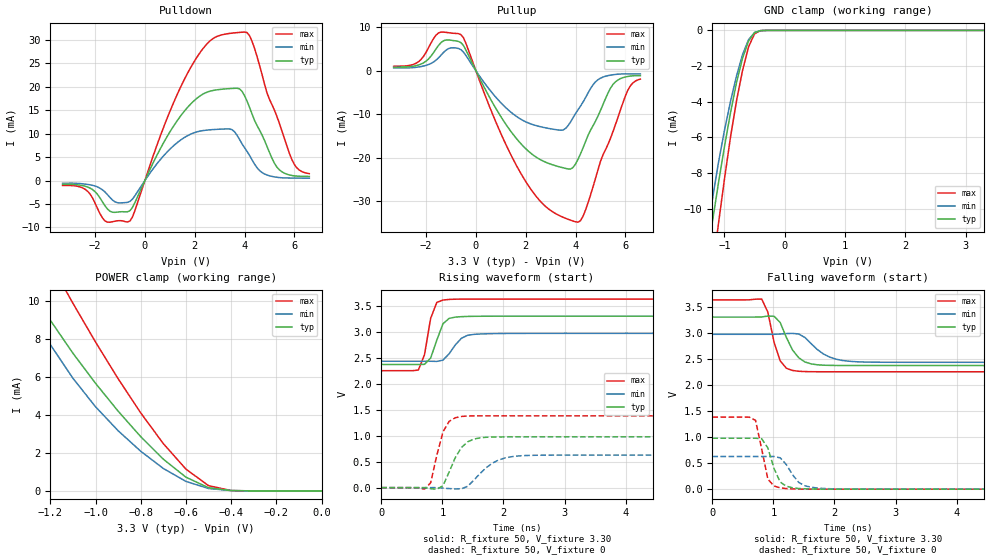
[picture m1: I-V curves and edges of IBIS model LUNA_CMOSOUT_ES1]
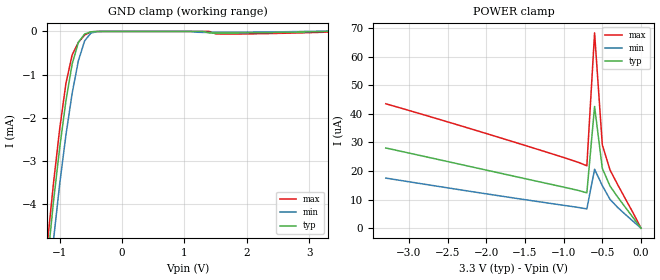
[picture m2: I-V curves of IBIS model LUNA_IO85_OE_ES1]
[IBIS Ver]   3.2
[Comment Char]   |_char
[File name]   sg-9101cga_33v_c.ibs
[File Rev]   1.0
[Date]   2017/11/24 16:18:06
[Source]
[Notes]
[Disclaimer]
This information is for modeling purposes only, and is not guaranteed.
Property of SEIKO EPSON Corp.,
unauthorized reproduction and/or distribution is strictly prohibited.
[Copyright]
Copyright 2017, SEIKO EPSON Corp.
[Component]   SG-9101CGA
Si_location Pin
Timing_location Pin
[Manufacturer]   SEIKO EPSON Corp.
| 2520 PKG
| 2520 PKG
[Package]
R_pkg   238m   NA   NA
L_pkg   2.1n   NA   NA
C_pkg   0.38p   NA   NA
[Pin] signal_name   model_name
1   OE   LUNA_IO85_OE_ES1
2   VSS   GND
3   OUT   LUNA_CMOSOUT_ES1
4   VDD   POWER
| Models and submodels in the file (2): LUNA_CMOSOUT_ES1 (3-state), LUNA_IO85_OE_ES1 (Input)
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[Model]   LUNA_CMOSOUT_ES1
Model_type 3-state
Enable Active-High
Polarity Non-Inverting
Vmeas=1.65
C_comp   2.5p   2.0p   3.0p
[Temperature Range] 25   105   -40
[Voltage Range]   3.30   2.97   3.63
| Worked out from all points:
|   slope of the pulldown table from 0 to 0.495 V, typ, clamps not added: 89.7 ohm
|   slope of the pullup table from 0 to 0.495 V, typ, clamps not added: 88.8 ohm
|   GND clamp passes 1 mA (typ) near -0.64 V on its own axis
|   POWER clamp passes 1 mA (typ) near -0.63 V on its own axis
|   falling waveform, R_fixture 50, V_fixture 3.30: 20-80 % time 249ps typ, 352ps min, 176ps max; typ from 3.3 V to 2.37 V
|   falling waveform, R_fixture 50, V_fixture 0: 20-80 % time 177ps typ, 233ps min, 148ps max; typ from 0.977 V to 0 V
|   rising waveform, R_fixture 50, V_fixture 3.30: 20-80 % time 170ps typ, 222ps min, 143ps max; typ from 2.37 V to 3.3 V
|   rising waveform, R_fixture 50, V_fixture 0: 20-80 % time 249ps typ, 369ps min, 183ps max; typ from 0 V to 0.977 V
[Pullup]
-3.3V     819.1uA    632.4uA    1.02mA
-2.3V     1.324mA    861.7uA    2.085mA
-1.5V     5.824mA    2.966mA    8.695mA
-600mV    6.462mA    4.844mA    8.302mA
900mV     -9.633mA   -6.754mA   -13.14mA
2V        -17.97mA   -11.78mA   -25.53mA
3.5V      -22.37mA   -13.65mA   -33.77mA
4.1V      -20.39mA   -8.97mA    -34.9mA
4.8V      -11.62mA   -2.566mA   -24.81mA
5.5V      -3.173mA   -932.8uA   -14.04mA
6.1V      -1.319mA   -729.2uA   -4.459mA
6.6V      -1.127mA   -733.5uA   -1.925mA
[Pulldown]
-3.3V     -797.7uA   -565.6uA   -1.043mA
-2.3V     -1.363mA   -809.2uA   -2.249mA
-1.6V     -5.373mA   -2.425mA   -8.597mA
-600mV    -6.419mA   -4.441mA   -8.617mA
900mV     9.459mA    6.142mA    13.38mA
2V        17.16mA    10.26mA    25.57mA
3.5V      19.66mA    10.86mA    31.46mA
4V        18.12mA    7.032mA    31.68mA
4.3V      14.22mA    4.45mA     29.74mA
5.3V      2.881mA    714uA      13.68mA
6V        1.012mA    547.6uA    3.442mA
6.6V      887.8uA    517.4uA    1.483mA
[GND Clamp]
-3.3V     -86.74mA   -76.76mA   -101.8mA
-1.3V     -13.11mA   -11.85mA   -16.24mA
-1.2V     -10.77mA   -9.503mA   -13.52mA
-1.1V     -8.591mA   -7.44mA    -10.88mA
-1V       -6.541mA   -5.623mA   -8.358mA
-900mV    -4.635mA   -4.001mA   -6.009mA
-800mV    -2.939mA   -2.563mA   -3.961mA
-700mV    -1.565mA   -1.365mA   -2.263mA
-600mV    -601.2uA   -521.6uA   -925.2uA
-500mV    -121.4uA   -116.4uA   -188.8uA
-300mV    -500.8nA   -1.29uA    -313.6nA
3.3V      193.1pA    4.095uA    131.4pA
[POWER Clamp]
-3.3V     73.68mA    63.39mA    89.04mA
-1.4V     13.2mA     11.93mA    16.56mA
-1.3V     10.93mA    9.714mA    14.21mA
-1.2V     8.97mA     7.69mA     11.99mA
-1.1V     7.236mA    5.92mA     9.861mA
-1V       5.655mA    4.424mA    7.824mA
-900mV    4.191mA    3.162mA    5.894mA
-700mV    1.665mA    1.179mA    2.483mA
-600mV    721.7uA    498.7uA    1.143mA
-500mV    167.2uA    126.9uA    275.1uA
-400mV    16.41uA    18.75uA    19.76uA
0V        193.1pA    1.068nA    160pA
[Falling Waveform]
R_fixture=50
V_fixture=3.30
V_fixture_min=2.97
V_fixture_max=3.63
0s        3.3V       2.97V      3.63V
808.1ps   3.303V     2.97V      3.646V
909.1ps   3.319V     2.97V      3.393V
1.01ns    3.316V     2.97V      2.819V
1.111ns   3.196V     2.975V     2.46V
1.313ns   2.668V     2.988V     2.276V
1.414ns   2.521V     2.976V     2.261V
1.919ns   2.374V     2.533V     2.251V
2.323ns   2.371V     2.446V     2.251V
10ns      2.371V     2.433V     2.251V
[Falling Waveform]
R_fixture=50
V_fixture=0
V_fixture_min=0
V_fixture_max=0
0s        977mV      626.2mV    1.382V
606.1ps   977mV      626.2mV    1.381V
707.1ps   977mV      626.2mV    1.32V
808.1ps   966.7mV    626.2mV    769.1mV
909.1ps   791mV      626.1mV    191.5mV
1.01ns    396.3mV    626.1mV    60.08mV
1.111ns   136.2mV    601.1mV    25.09mV
1.414ns   13.47mV    129.7mV    2.178mV
1.818ns   1.046mV    13.56mV    64.51uV
10ns      0V         0V         0V
[Rising Waveform]
R_fixture=50
V_fixture=3.30
V_fixture_min=2.97
V_fixture_max=3.63
0s        2.371V     2.433V     2.251V
606.1ps   2.371V     2.433V     2.263V
707.1ps   2.373V     2.433V     2.558V
808.1ps   2.494V     2.433V     3.26V
909.1ps   2.842V     2.43V      3.566V
1.01ns    3.156V     2.455V     3.611V
1.111ns   3.258V     2.578V     3.623V
1.313ns   3.291V     2.876V     3.629V
1.616ns   3.299V     2.958V     3.63V
10ns      3.3V       2.97V      3.63V
[Rising Waveform]
R_fixture=50
V_fixture=0
V_fixture_min=0
V_fixture_max=0
0s        0V         0V         0V
707.1ps   -1.034mV   -39nV      -27.85mV
808.1ps   -21.15mV   34.76uV    92.61mV
1.01ns    36.75mV    -8.306mV   1.074V
1.111ns   301.4mV    -18.63mV   1.276V
1.313ns   774.2mV    -23.09mV   1.37V
1.515ns   934.4mV    143.8mV    1.381V
1.818ns   974.1mV    470.8mV    1.382V
2.323ns   977mV      616.4mV    1.382V
10ns      977mV      626.2mV    1.382V
[Ramp]
R_load=50
dV/dt_r   5.862E-1/2.483E-10   3.757E-1/3.642E-10   8.295E-1/1.825E-10
dV/dt_f   5.572E-1/2.451E-10   3.223E-1/3.470E-10   8.273E-1/1.713E-10
|[End   LUNA_CMOSOUT_ES1
[Model]   LUNA_IO85_OE_ES1
Model_type Input
Enable Active-Low
Polarity Non-Inverting
Vinh=2.55
Vinl=0.89
C_comp   2.5p   2.0p   3.0p
[Temperature Range] 25   105   -40
[Voltage Range]   3.30   2.97   3.63
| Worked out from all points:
|   GND clamp passes 1 mA (typ) near -0.83 V on its own axis
[GND Clamp]
-3.3V     -49.97mA   -47.74mA   -53.94mA
-1.2V     -5.408mA   -6.351mA   -4.953mA
-1.1V     -3.959mA   -4.854mA   -3.533mA
-1V       -2.702mA   -3.543mA   -2.264mA
-900mV    -1.612mA   -2.406mA   -1.207mA
-800mV    -755.8uA   -1.435mA   -544.3uA
-700mV    -251.9uA   -680.1uA   -254.3uA
-600mV    -60.6uA    -218.5uA   -85.08uA
-500mV    -8.506uA   -39.85uA   -10.99uA
-400mV    -1.005uA   -4.241uA   -1.145uA
1.7V      -37.51uA   -20.16uA   -61.79uA
3.3V      135.9pA    8.008uA    -15.73uA
[POWER Clamp]
-3.3V     28.08uA    17.53uA    43.56uA
-1.6V     17.94uA    10.38uA    29.81uA
-900mV    13.77uA    7.613uA    23.86uA
-700mV    12.37uA    6.737uA    21.84uA
-600mV    42.62uA    20.63uA    68.38uA
-500mV    20.91uA    14.89uA    29.15uA
-400mV    14.72uA    10.06uA    20.36uA
-300mV    10.84uA    7.224uA    15.17uA
-100mV    3.62uA     2.354uA    5.264uA
0V        135.7pA    303.7pA    135.4pA
